DATA_BLOCK "DIVE_DB"
TITLE =
VERSION : 0.1


  STRUCT
   RUN : BOOL ;	//Produzione in corso
   MANUALE : BOOL ;	//Manuale
   ALLARME : BOOL ;	//Allarme
   MANCATO_CARICO : BOOL ;	//Mancato Carico
   MANCATO_SCARICO : BOOL ;	//Mancato Scarico
   PRESENZA_PEZZO : BOOL ;	//Presenza pezzo
   ESITO_OK : BOOL ;	//Pezzo OK
   ESITO_KO : BOOL ;	//Pezzo KO
   COMANDO_BARRA2_AVANTI : BOOL ;
   FINE_LAVORO : BOOL ;	//Lavorazione finita
   INIZIO_PALLET : BOOL ;	//Inizio pallet
   FINE_PALLET : BOOL ;	//Fine pallet
   PEZZI_BUONI : BOOL ;	//Segnale pezzo buono
   PEZZI_SCARTO : BOOL ;	//Segnale pezzo scarto
   COMANDO_BARRA1_AVANTI : BOOL ;	//Disponibile
   LIFE : BOOL ;	//Disponibile
   CODICE_PALLET : DWORD ;	//Numero codice pallet
   SPARE_DWORD_1 : DWORD ;	//Disponibile
   SPARE_DWORD_2 : DWORD ;	//Disponibile
   SCARTO : BOOL ;	//Pezzo Scarto
   SPARE1 : BOOL ;	//Disponibile
   SPARE2 : BOOL ;	//Disponibile
   SPARE3 : BOOL ;	//Disponibile
   SPARE4 : BOOL ;	//Disponibile
   SPARE5 : BOOL ;	//Disponibile
   SPARE6 : BOOL ;	//Disponibile
   SPARE7 : BOOL ;	//Disponibile
   SPARE8 : BOOL ;	//Disponibile
   SPARE9 : BOOL ;	//Disponibile
   SPARE10 : BOOL ;	//Disponibile
   SPARE11 : BOOL ;	//Disponibile
   SPARE12 : BOOL ;	//Disponibile
   SPARE13 : BOOL ;	//Disponibile
   SPARE14 : BOOL ;	//Disponibile
   SPARE15 : BOOL ;	//Disponibile
   SPARE_DWORD_3 : DWORD ;	//Disponibile
   SPARE_DWORD_4 : DWORD ;	//Disponibile
  END_STRUCT ;
BEGIN
   RUN := FALSE;
   MANUALE := FALSE;
   ALLARME := FALSE;
   MANCATO_CARICO := FALSE;
   MANCATO_SCARICO := FALSE;
   PRESENZA_PEZZO := FALSE;
   ESITO_OK := FALSE;
   ESITO_KO := FALSE;
   COMANDO_BARRA2_AVANTI := FALSE;
   FINE_LAVORO := FALSE;
   INIZIO_PALLET := FALSE;
   FINE_PALLET := FALSE;
   PEZZI_BUONI := FALSE;
   PEZZI_SCARTO := FALSE;
   COMANDO_BARRA1_AVANTI := FALSE;
   LIFE := FALSE;
   CODICE_PALLET := DW#16#0;
   SPARE_DWORD_1 := DW#16#0;
   SPARE_DWORD_2 := DW#16#0;
   SCARTO := FALSE;
   SPARE1 := FALSE;
   SPARE2 := FALSE;
   SPARE3 := FALSE;
   SPARE4 := FALSE;
   SPARE5 := FALSE;
   SPARE6 := FALSE;
   SPARE7 := FALSE;
   SPARE8 := FALSE;
   SPARE9 := FALSE;
   SPARE10 := FALSE;
   SPARE11 := FALSE;
   SPARE12 := FALSE;
   SPARE13 := FALSE;
   SPARE14 := FALSE;
   SPARE15 := FALSE;
   SPARE_DWORD_3 := DW#16#0;
   SPARE_DWORD_4 := DW#16#0;
END_DATA_BLOCK

